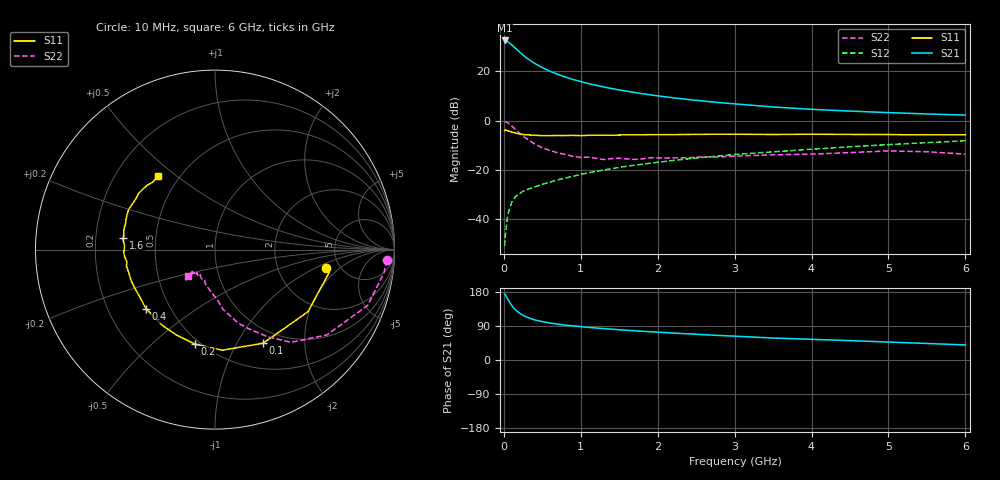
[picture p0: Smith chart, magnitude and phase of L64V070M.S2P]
!  INFINEON TECHNOLOGIES Small Signal Semiconductors
! BFR380L3 , Si-NPN RF-Transistor in TSLP-3-1
!  Vce=4 V,  Ic=70 mA
! Common Emitter S-Parameters:  07. March 2005
#  GHz  S  MA  R  50
! f  S11  S21  S12  S22
! GHz  Mag  Ang  Mag  Ang  Mag  Ang  Mag  Ang
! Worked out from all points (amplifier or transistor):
!   36 points, 10 MHz to 6 GHz, reference 50 ohm
!   highest |S21| = 32.6 dB at 10 MHz (marker M1)
!   |S21| within 3 dB of that: start of sweep to 145.5 MHz
!   unconditionally stable (mu >= 1): 1.388 GHz to 4.823 GHz
!   at 250 MHz: K = 0.50, MSG = 27.7 dB, |S12| = -28.7 dB
!   at 1.4 GHz: K = 1.00, MAG = 16.1 dB, |S12| = -19.6 dB
!   at 6 GHz: K = 0.97, MSG = 5.2 dB, |S12| = -8.2 dB
!   S11 on the Smith chart (normalised r, x): 10 MHz: 3.90, -1.34; 100 MHz: 0.81, -1.29; 200 MHz: 0.47, -0.69; 400 MHz: 0.37, -0.33; 1.6 GHz: 0.32, +0.05; 6 GHz: 0.39, +0.43
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0.01  0.629 -9.5  42.76 174.3  0.0028 72.6  0.9595 -3.5
0.02  0.6487 -11.4  42.38 172.3  0.0047 86.8  0.9497 -8.0
0.05  0.6229 -33.8  40.55 160.5  0.012 77.0  0.9054 -20.1
0.1  0.5867 -62.8  35.22 144.6  0.0217 65.4  0.7841 -37.3
0.15  0.562 -85.9  29.81 132.5  0.0284 59.5  0.6676 -50.7
0.2  0.538 -102.1  25.14 124.0  0.0326 57.4  0.5668 -58.9
0.25  0.5215 -114.9  21.57 117.8  0.0366 54.1  0.4792 -67.0
0.3  0.5139 -124.7  18.66 112.9  0.0394 55.4  0.4268 -72.7
0.4  0.5063 -139.2  14.67 105.9  0.0449 54.9  0.3353 -82.4
0.5  0.4952 -148.4  12.01 101.3  0.051 57.0  0.28 -87.3
0.6  0.4962 -155.4  10.09 97.6  0.056 58.5  0.2477 -93.0
0.7  0.4983 -160.3  8.753 94.7  0.0625 60.3  0.2217 -98.6
0.9  0.502 -169.7  6.867 90.0  0.0738 62.5  0.1871 -108.0
1.1  0.5043 -175.2  5.681 86.1  0.087 64.3  0.1804 -113.3
1.3  0.5056 179.2  4.85 82.8  0.0998 65.6  0.162 -120.4
1.6  0.5162 173.0  3.959 78.4  0.1183 66.3  0.166 -128.1
2.2  0.5192 163.7  2.92 71.1  0.1548 67.0  0.1747 -130.1
2.8  0.5308 155.2  2.333 64.8  0.1912 66.8  0.1827 -136.4
3.5  0.5237 147.0  1.898 58.0  0.2322 64.6  0.2021 -135.0
4.5  0.5249 140.9  1.564 51.1  0.294 62.9  0.2239 -134.3
5.5  0.5122 132.7  1.368 43.6  0.3573 59.1  0.233 -133.9
6  0.5167 127.7  1.297 39.8  0.3901 56.9  0.2085 -135.6
